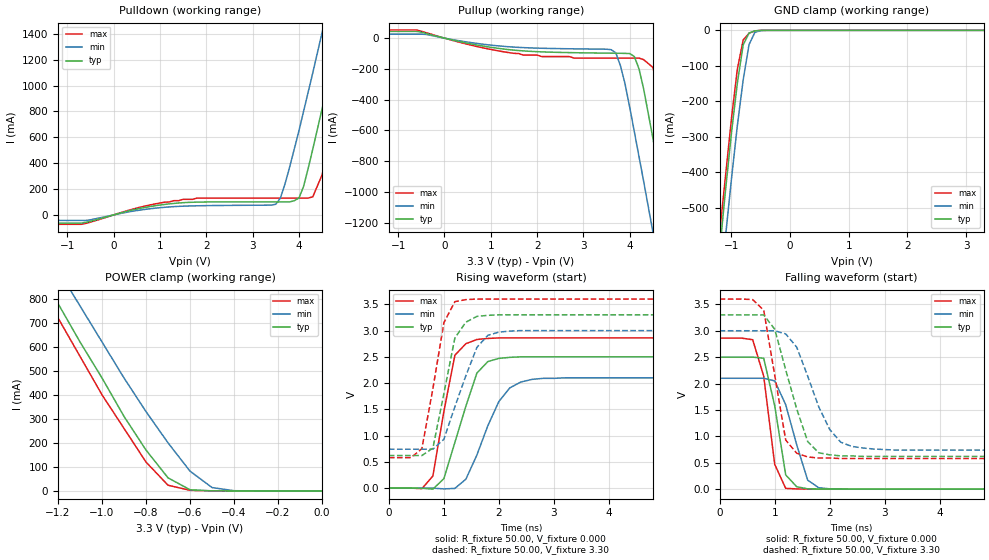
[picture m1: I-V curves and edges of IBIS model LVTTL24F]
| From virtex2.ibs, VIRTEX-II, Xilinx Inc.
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|   Model LVTTL24F
[Model]   LVTTL24F
Model_type   I/O
Polarity   Non-Inverting
Enable   Active-Low
Vinh = 2.0V
Vinl = 0.8V
Vmeas =   1.40V
Cref =  35.00pF
Rref =   1.00M
Vref =  0.000V
C_comp   7.00pF   6.00pF   8.00pF
[Temperature Range]   25.00   100.00   0.000
[Voltage Range]   3.30V   3.00V   3.60V
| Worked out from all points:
|   slope of the pulldown table from 0 to 0.495 V, typ, clamps not added: 11.1 ohm
|   slope of the pullup table from 0 to 0.495 V, typ, clamps not added: 15 ohm
|   GND clamp passes 1 mA (typ) near -0.57 V on its own axis
|   POWER clamp passes 1 mA (typ) near -0.52 V on its own axis
|   rising waveform, R_fixture 50.00, V_fixture 0.000: 20-80 % time 447ps typ, 514ps min, 299ps max; typ from 0 V to 2.5 V
|   rising waveform, R_fixture 50.00, V_fixture 3.30: 20-80 % time 306ps typ, 467ps min, 299ps max; typ from 0.62 V to 3.3 V
|   falling waveform, R_fixture 50.00, V_fixture 0.000: 20-80 % time 258ps typ, 361ps min, 231ps max; typ from 2.5 V to 0 V
|   falling waveform, R_fixture 50.00, V_fixture 3.30: 20-80 % time 448ps typ, 520ps min, 295ps max; typ from 3.3 V to 0.62 V
[Pulldown]
| voltage   I(typ)   I(min)   I(max)
-3.3V     -63.55mA   -42.85mA   -72.72mA
-700mV    -63.55mA   -42.85mA   -72.64mA
1.5V      94.54mA    67.4mA     120mA
3.5V      100mA      82mA       130mA
3.7V      100mA      240mA      130mA
4V        130mA      650mA      130mA
4.3V      510mA      1.1A       140mA
4.5V      820mA      1.41A      310mA
4.9V      1.47A      2.04A      930mA
5.1V      1.79A      2.35A      1.25A
5.3V      2.12A      2.67A      1.58A
6.6V      4.29A      4.73A      3.74A
[Pullup]
| voltage   I(typ)   I(min)   I(max)
-3.3V     43.55mA    25.59mA    52.52mA
-600mV    43.55mA    25.59mA    52.52mA
1.7V      -83mA      -61.63mA   -110mA
3.6V      -97.83mA   -75.1mA    -130mA
3.8V      -98.45mA   -180mA     -130mA
4V        -100mA     -450mA     -130mA
4.2V      -200mA     -770mA     -130mA
4.5V      -650mA     -1.26A     -190mA
4.9V      -1.33A     -1.93A     -780mA
5.1V      -1.68A     -2.27A     -1.12A
5.3V      -2.03A     -2.62A     -1.47A
6.6V      -4.33A     -4.85A     -3.76A
[GND_clamp]
| voltage   I(typ)   I(min)   I(max)
-3.3V     -4.3A      -4.31A     -4.26A
-1.2V     -620mA     -740mA     -570mA
-1.1V     -450mA     -580mA     -410mA
-1V       -290mA     -420mA     -250mA
-900mV    -150mA     -270mA     -110mA
-800mV    -41.03mA   -140mA     -27.28mA
-700mV    -7.6mA     -40.21mA   -8.18mA
-600mV    -1.42mA    -5.61mA    -1.62mA
-500mV    -130uA     -670uA     -130uA
3.3V      67.85pA    43.48uA    45.6pA
[POWER_clamp]
| voltage   I(typ)   I(min)   I(max)
-3.3V     4.25A      4.22A      4.2A
-1.3V     940mA      1.07A      880mA
-1.2V     780mA      920mA      720mA
-1.1V     620mA      770mA      560mA
-1V       470mA      620mA      400mA
-900mV    310mA      470mA      260mA
-800mV    170mA      330mA      120mA
-700mV    54.34mA    200mA      23.62mA
-600mV    4.76mA     82.21mA    2.52mA
-500mV    280uA      14.02mA    260uA
-400mV    16.9uA     860uA      14.85uA
0V        67.85pA    2.04nA     61.89pA
[Ramp]
| variable   typ   min   max
dV/dt_r   1.50/0.35n   1.26/0.49n   1.72/0.28n
dV/dt_f   1.61/0.36n   1.36/0.50n   1.81/0.28n
R_load = 50.00
[Rising Waveform]
R_fixture = 50.00
V_fixture = 0.000
| time   V(typ)   V(min)   V(max)
0s        0V         0V         0V
600ps     -2.97mV    49.64uV    -11.25mV
800ps     -20.34mV   -1.44mV    230mV
1ns       180mV      -15.18mV   1.46V
1.2ns     870mV      -6.11mV    2.53V
1.4ns     1.56V      170mV      2.75V
1.6ns     2.19V      630mV      2.83V
2ns       2.47V      1.65V      2.86V
2.6ns     2.5V       2.07V      2.86V
10ns      2.5V       2.1V       2.86V
[Rising Waveform]
R_fixture = 50.00
V_fixture = 3.30
V_fixture_min = 3.00
V_fixture_max = 3.60
| time   V(typ)   V(min)   V(max)
0s        620mV      740mV      580mV
400ps     620mV      740mV      580mV
600ps     620mV      740mV      750mV
800ps     760mV      740mV      1.89V
1ns       1.8V       930mV      3.15V
1.2ns     2.86V      1.55V      3.55V
1.4ns     3.16V      2.14V      3.59V
1.6ns     3.27V      2.68V      3.6V
2ns       3.3V       2.97V      3.6V
10ns      3.3V       3V         3.6V
[Falling Waveform]
R_fixture = 50.00
V_fixture = 0.000
| time   V(typ)   V(min)   V(max)
0s        2.5V       2.1V       2.86V
600ps     2.5V       2.1V       2.83V
800ps     2.48V      2.1V       2.14V
1ns       1.58V      2.05V      470mV
1.2ns     270mV      1.6V       15.47mV
1.4ns     46.28mV    840mV      4.58mV
1.6ns     5.98mV     170mV      1.53mV
1.8ns     2.03mV     27.59mV    650uV
2.4ns     270uV      1.35mV     74.53uV
10ns      -6.22uV    -1.45uV    -3.02uV
[Falling Waveform]
R_fixture = 50.00
V_fixture = 3.30
V_fixture_min = 3.00
V_fixture_max = 3.60
| time   V(typ)   V(min)   V(max)
0s        3.3V       3V         3.6V
600ps     3.3V       3V         3.59V
800ps     3.3V       3V         3.39V
1ns       3.03V      3V         2.16V
1.2ns     2.26V      2.94V      930mV
1.4ns     1.52V      2.69V      680mV
1.6ns     900mV      2.14V      610mV
2ns       650mV      1.13V      590mV
2.4ns     630mV      810mV      580mV
10ns      620mV      740mV      580mV
